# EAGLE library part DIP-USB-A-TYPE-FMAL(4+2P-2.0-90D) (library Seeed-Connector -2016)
320010007
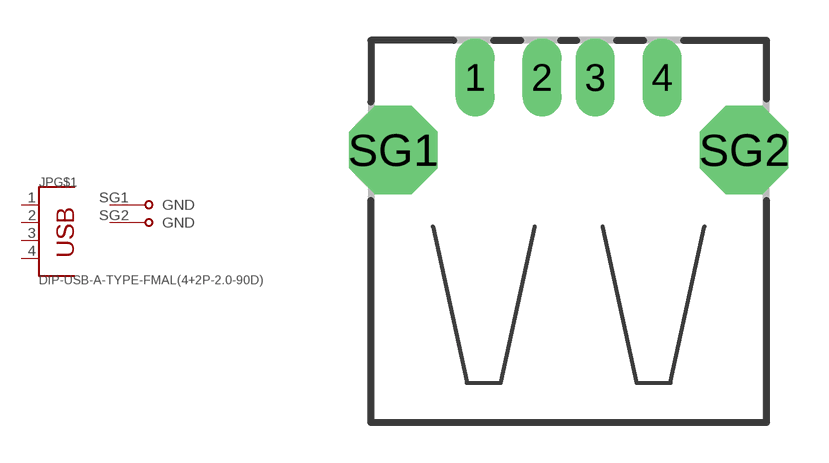
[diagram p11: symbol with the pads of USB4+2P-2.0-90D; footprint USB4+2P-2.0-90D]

Designator prefix JP; gates G$1=ST-USB-003A G$2=SGND G$3=SGND

## DIP-USB-A-TYPE-FMAL(4+2P-2.0-90D) (VALUE: USB4-2.0-90D)  [USB4+2P-2.0-90D]
1  G$1:1
2  G$1:2
3  G$1:3
4  G$1:4
SG1  G$2:GND  pas
SG2  G$3:GND  pas

## Footprint USB4+2P-2.0-90D (pad centres in mm)
USB connector
drill 0.95 long: 1 -3.5,2.71; 2 -1,2.71; 3 1,2.71; 4 3.5,2.71
drill 2.3 octagon: SG1 -6.57,0; SG2 6.57,0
